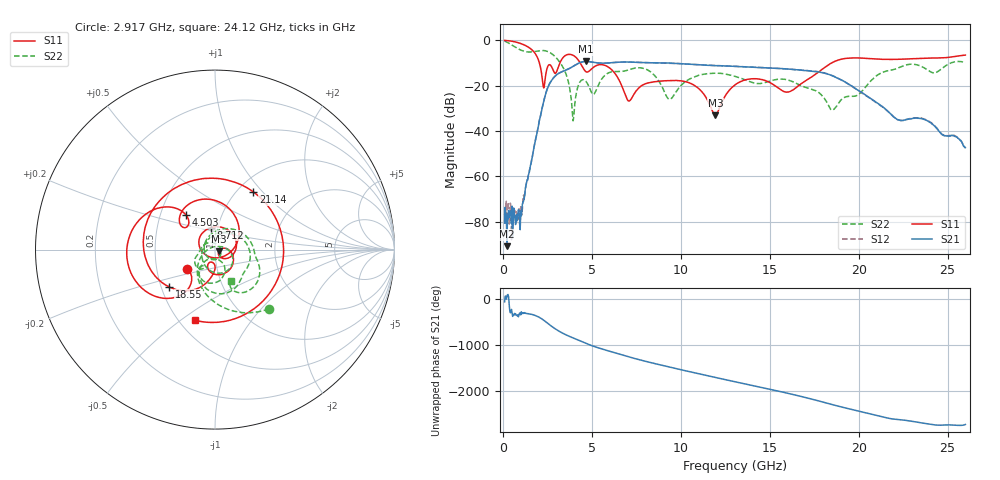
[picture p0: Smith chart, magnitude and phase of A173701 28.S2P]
!  2-Port S-parameters saved by WinCal
! VAR MeasName=S-Parameters (CALIBRATED_DATA) read from VNA (N5245A)
! VAR MeasDate=2017-6-7 10:30:13
! VAR NAME=A173701 28
! VAR FILENAME=A173701 28.S2P
! VAR DATE=2017-6-7 10:30:13
! VAR PHYS_PORTS=1,2
# Hz S DB R 50
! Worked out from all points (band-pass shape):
!   801 points, 100 MHz to 26 GHz, reference 50 ohm
!   highest |S21| = -9.27 dB at 4.665 GHz (marker M1); lowest = -90.8 dB at 229.5 MHz (marker M2)
!   |S21| within 3 dB of the highest: 3.766 GHz to 15.3 GHz (11.54 GHz wide, 121 % of centre)
!   lowest |S11| = -33.0 dB at 11.95 GHz (marker M3), VSWR 1.05, Z = 52.1 - j0.922 ohm
!   |S11| at or under -10 dB: 2.057 GHz to 3.205 GHz (1.147 GHz wide, 43.6 % of centre); 4.353 GHz to 18.47 GHz (14.11 GHz wide, 124 % of centre)
!   |S22| runs from -35.5 to -0.3 dB; largest |S21 - S12| = 0.0041
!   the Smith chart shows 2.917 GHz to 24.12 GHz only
!   S11 on the Smith chart (normalised r, x): 2.917 GHz: 0.72, -0.16; 4.503 GHz: 0.68, +0.28; 8.712 GHz: 0.93, +0.23; 18.55 GHz: 0.55, -0.26; 21.14 GHz: 1.18, +0.89; 24.12 GHz: 0.60, -0.57
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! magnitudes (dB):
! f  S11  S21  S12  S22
! 100 MHz  0.0  -80.6  -76.5  -0.3
! 229.5 MHz  -0.1  -90.8  -82.4  -0.7
! 974.1 MHz  -1.3  -83.5  -83.2  -4.1
! 2.301 GHz  -21.0  -26.8  -26.8  -4.5
! 2.917 GHz  -14.4  -15.9  -15.9  -7.0
! 3.953 GHz  -6.6  -11.4  -11.4  -35.5
! 4.438 GHz  -11.2  -9.5  -9.5  -17.5
! 4.503 GHz  -12.1  -9.4  -9.4  -17.3
! 4.665 GHz  -13.8  -9.3  -9.3  -18.0
! 5.928 GHz  -11.7  -10.0  -10.0  -14.4
! 7.093 GHz  -26.7  -9.6  -9.5  -12.9
! 8.712 GHz  -18.1  -9.9  -9.9  -17.3
! 8.744 GHz  -18.0  -9.9  -9.9  -17.7
! 9.392 GHz  -17.7  -10.0  -10.0  -25.9
! 11.95 GHz  -33.0  -11.1  -11.1  -14.4
! 13.05 GHz  -19.6  -11.4  -11.5  -15.9
! 17.39 GHz  -16.0  -13.6  -13.5  -21.6
! 18.55 GHz  -9.6  -15.7  -15.6  -30.7
! 21.14 GHz  -8.3  -28.1  -28.2  -14.9
! 21.69 GHz  -8.4  -31.6  -31.7  -13.3
! 24.12 GHz  -7.8  -36.9  -36.5  -14.2
! 26 GHz  -6.5  -47.3  -47.3  -9.9
